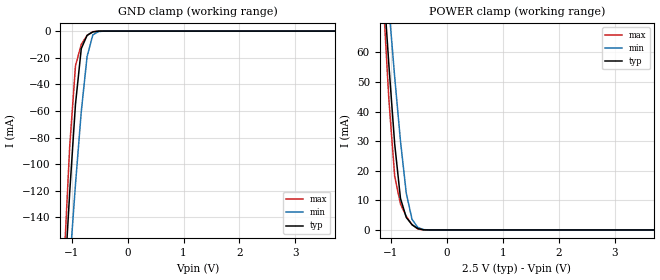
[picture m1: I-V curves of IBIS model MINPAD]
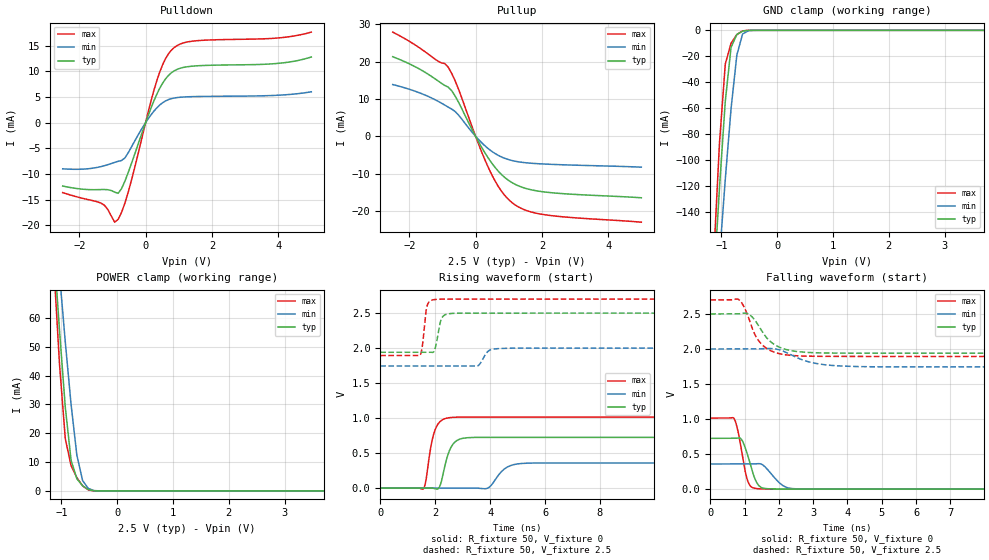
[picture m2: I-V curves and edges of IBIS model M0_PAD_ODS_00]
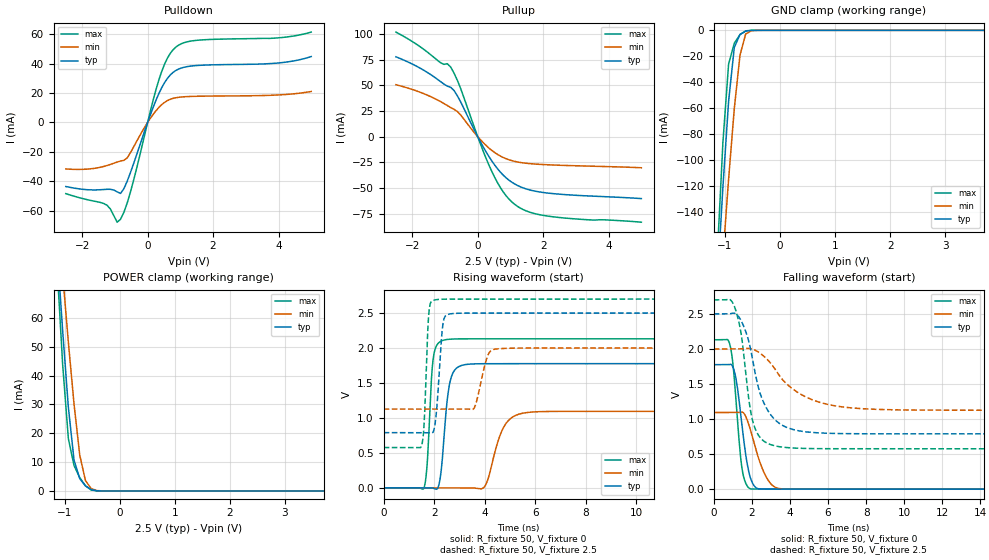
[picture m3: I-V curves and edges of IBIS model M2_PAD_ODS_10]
| Created by SiliconSmart  S-2021.06-SP5-2
[IBIS Ver]   4.0
[File Name]   as320ck_25v_rev1p1.ibs
[File Rev]   1.1
[Date]   Tue Aug 20 2024
|[Source]   Avalanche Team
|[Notes]   Generated IBIS models from Silicon Smart
|[Rev 1.0]   Initial release based on extracted netlist
|[Rev 1.1]   Updated the VCC supply values according to
|		datasheet
|[Disclaimer]   THE MODEL LIBRARIES ARE PROVIDED AS IS.
|[Copyright]   Copyright 2024, Avalanche Technology, All Rights Reserved
[Component]   AS30XX20X_BGA
[Manufacturer]  Avalanche Technology
| CONTENT :
| This file contains IBIS MODEL for PSRAM device
| AS30XX20X
| USAGE :
| The models are derived for the 2.0V to 2.7V I/O Operation.
| Temperatures for model generation: typ: 25, max: -40, min: 125
| Voltages : typ: 2.5V, min: 2.0V, max: 2.7V
| PACKAGES SUPPORTED :
| 56-ball FBGA (10mm x 10mm)
| VERIFICATION
| Errors  : 0
| Warnings: 11
| All warnings due to non-monotonic data:
[Package]
|  Design die-package: BGA
| variable   typ   min   max
R_pkg   0.72029   0.51528   1.0002
L_pkg   5.797e-9   4.155e-9   8.073e-9
C_pkg   1.116e-12   7.907e-13   1.753e-12
|Pin and Model info
[Pin]  signal_name  model_name   R_pin   L_pin   C_pin
E2   CS1#   MINPAD   0.4340	15.2000E-9	1.2600E-12
C3   CS2#   MINPAD   0.3800	13.5000E-9	1.0400E-12
D2   CLK1   MINPAD   0.4300	12.7000E-9	0.9790E-12
D1   CLK2   MINPAD   0.4480	14.6000E-9	1.1600E-12
F3   IO_0   MIOPAD   0.4010	12.4000E-9	1.2500E-12
F2   IO_1   MIOPAD   0.4050	14.2000E-9	1.1100E-12
E4   IO_2   MIOPAD   0.3780	11.8000E-9	1.2000E-12
F4   IO_3   MIOPAD   0.3700	11.8000E-9	1.2600E-12
F5   IO_4   MIOPAD   0.3710	11.1000E-9	1.1000E-12
G3   IO_5   MIOPAD   0.4050	13.8000E-9	1.1600E-12
G2   IO_6   MIOPAD   0.3830	15.2000E-9	1.0900E-12
G1   IO_7   MIOPAD   0.4480	16.4000E-9	1.0800E-12
C7   HTBSEL   MINPAD   0.1380	6.1700E-9	0.6060E-12
B7   HBP_2   MINPAD   0.1470	6.3900E-9	1.0000E-12
A6   HBP_1   MINPAD   0.1910	8.5000E-9	1.1500E-12
A5   HBP_0   MINPAD   0.2050	8.6800E-9	1.4200E-12
C4   RESET#   MINPAD   0.3410	14.1000E-9	1.6300E-12
C5   INT1#   MIOPAD   0.3080	12.5000E-9	1.2100E-12
D3   INT2#   MIOPAD   0.2120	10.3000E-9	0.8230E-12
B1   VSSIO   GND   NA   NA   NA
B5   VSSIO   GND   NA   NA   NA
B6   VSSIO   GND   NA   NA   NA
E1   VSSIO   GND   NA   NA   NA
G5   VSSIO   GND   NA   NA   NA
G6   VSSIO   GND   NA   NA   NA
A1   VSS   GND   NA   NA   NA
A3   VSS   GND   NA   NA   NA
B3   VSS   GND   NA   NA   NA
E5   VSS   GND   NA   NA   NA
E6   VSS   GND   NA   NA   NA
E7   VSS   GND   NA   NA   NA
G7   VSS   GND   NA   NA   NA
A8   VSS   GND   NA   NA   NA
A7   VCCIO   POWER   NA   NA   NA
B2   VCCIO   POWER   NA   NA   NA
B4   VCCIO   POWER   NA   NA   NA
C6   VCCIO   POWER   NA   NA   NA
F1   VCCIO   POWER   NA   NA   NA
F6   VCCIO   POWER   NA   NA   NA
G4   VCCIO   POWER   NA   NA   NA
A2   VCC   POWER   NA   NA   NA
A4   VCC   POWER   NA   NA   NA
D4   VCC   POWER   NA   NA   NA
D6   VCC   POWER   NA   NA   NA
D7   VCC   POWER   NA   NA   NA
F7   VCC   POWER   NA   NA   NA
| IOPAD
[Model Selector] MIOPAD
| Model Description
M0_PAD_ODS_00   35ohms
M1_PAD_ODS_01   40ohms
M2_PAD_ODS_10   20ohms
M3_PAD_ODS_11   15ohms
| Models and submodels in the file (5): MINPAD (Input), M0_PAD_ODS_00 (I/O), M2_PAD_ODS_10 (I/O), M1_PAD_ODS_01 (I/O), M3_PAD_ODS_11 (I/O)
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[Model] MINPAD
Model_type Input
Enable   Active-High
Vinl  =  0.7
Vinh  =  1.8
| Capacitance  typ   min   max
C_comp   1.561946e-12   1.465732e-12   1.706605e-12
| Variables   typ   min   max
[GND Clamp Reference]   0   0   0
[POWER Clamp Reference]   2.5   2   2.7
[Pulldown Reference]   0   0   0
[Pullup Reference]   2.5   2   2.7
[Temperature Range]   25   125   -40
[Voltage Range]   2.5   2   2.7
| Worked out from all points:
|   GND clamp passes 1 mA (typ) near -0.64 V on its own axis
|   POWER clamp passes 1 mA (typ) near -0.56 V on its own axis
[GND Clamp]
| Voltage   I(typ)   I(min)   I(max)
-2.5V     -1.297A    -1.146A    -1.538A
-1.138V   -195.9mA   -238.3mA   -175.2mA
-1.034V   -121.2mA   -175.1mA   -86.57mA
-931mV    -54.79mA   -114.9mA   -26.01mA
-827.6mV  -13.15mA   -60.41mA   -9.964mA
-724.1mV  -3.204mA   -19.15mA   -3.279mA
-620.7mV  -615.2uA   -2.798mA   -407.3uA
-517.2mV  -34.38uA   -319.4uA   -6.503uA
-413.8mV  -821.1nA   -24.43uA   -50.87nA
5V        0A         0A         0A
[POWER Clamp]
| Voltage   I(typ)   I(min)   I(max)
-2.5V     511mA      454.9mA    606.6mA
-1.138V   84.76mA    99.9mA     78.64mA
-1.034V   55.67mA    75.27mA    43.94mA
-931mV    29.07mA    51.7mA     18.16mA
-827.6mV  10.68mA    30.08mA    8.788mA
-724.1mV  4.238mA    12.45mA    4.618mA
-620.7mV  1.771mA    3.587mA    1.776mA
-517.2mV  465uA      837.9uA    329.7uA
-413.8mV  47.65uA    120.2uA    11.19uA
-310.3mV  1.515uA    11.72uA    116.8nA
5V        0A         0A         0A
[Model] M0_PAD_ODS_00
Model_type I/O
Enable   Active-High
Vinl  =  0.7
Vinh  =  1.8
Vmeas =  1.25
Cref  =  30e-12
| Capacitance  typ   min   max
C_comp   1.568193e-12   1.472592e-12   1.715469e-12
| Variables   typ   min   max
[GND Clamp Reference]   0   0   0
[POWER Clamp Reference]   2.5   2   2.7
[Pulldown Reference]   0   0   0
[Pullup Reference]   2.5   2   2.7
[Temperature Range]   25   125   -40
[Voltage Range]   2.5   2   2.7
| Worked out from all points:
|   slope of the pulldown table from 0 to 0.375 V, typ, clamps not added: 62.2 ohm
|   slope of the pullup table from 0 to 0.375 V, typ, clamps not added: 65.7 ohm
|   GND clamp passes 1 mA (typ) near -0.64 V on its own axis
|   POWER clamp passes 1 mA (typ) near -0.56 V on its own axis
|   falling waveform, R_fixture 50, V_fixture 0: 20-80 % time 278ps typ, 405ps min, 227ps max; typ from 0.725 V to 0 V
|   falling waveform, R_fixture 50, V_fixture 2.5: 20-80 % time 573ps typ, 848ps min, 480ps max; typ from 2.5 V to 1.94 V
|   rising waveform, R_fixture 50, V_fixture 0: 20-80 % time 317ps typ, 472ps min, 280ps max; typ from 0 V to 0.725 V
|   rising waveform, R_fixture 50, V_fixture 2.5: 20-80 % time 165ps typ, 246ps min, 130ps max; typ from 1.94 V to 2.5 V
[GND Clamp]
| Voltage   I(typ)   I(min)   I(max)
-2.5V     -1.297A    -1.146A    -1.538A
-1.138V   -195.9mA   -238.3mA   -175.2mA
-1.034V   -121.2mA   -175.1mA   -86.57mA
-931mV    -54.79mA   -114.9mA   -26.01mA
-827.6mV  -13.15mA   -60.41mA   -9.967mA
-724.1mV  -3.205mA   -19.15mA   -3.28mA
-620.7mV  -615.3uA   -2.798mA   -407.6uA
-517.2mV  -34.39uA   -319.4uA   -6.513uA
-413.8mV  -821.3nA   -24.43uA   -50.96nA
5V        0A         0A         0A
[POWER Clamp]
| Voltage   I(typ)   I(min)   I(max)
-2.5V     511mA      454.9mA    606.6mA
-1.138V   84.76mA    99.9mA     78.64mA
-1.034V   55.67mA    75.27mA    43.94mA
-931mV    29.07mA    51.7mA     18.16mA
-827.6mV  10.68mA    30.08mA    8.788mA
-724.1mV  4.238mA    12.45mA    4.618mA
-620.7mV  1.771mA    3.587mA    1.776mA
-517.2mV  465uA      837.9uA    329.7uA
-413.8mV  47.65uA    120.2uA    11.19uA
-310.3mV  1.515uA    11.72uA    116.8nA
5V        0A         0A         0A
[Pulldown]
| Voltage   I(typ)   I(min)   I(max)
-2.5V     -12.37mA   -9.009mA   -13.66mA
-1.345V   -13.05mA   -8.574mA   -15.7mA
-1.138V   -13.09mA   -8.194mA   -16.96mA
-931mV    -13.56mA   -7.743mA   -19.43mA
-827.6mV  -13.79mA   -7.541mA   -18.86mA
-517.2mV  -9.616mA   -5.796mA   -13.4mA
344.8mV   5.633mA    2.926mA    8.322mA
603.4mV   8.558mA    4.247mA    12.51mA
948.3mV   10.39mA    4.896mA    15.04mA
1.638V    11.13mA    5.111mA    16.04mA
3.99V     11.57mA    5.352mA    16.53mA
5V        12.82mA    6.029mA    17.68mA
[Pullup]
| Voltage   I(typ)   I(min)   I(max)
-2.5V     21.32mA    13.87mA    27.92mA
-1.552V   17.3mA     11.16mA    22.82mA
-827.6mV  13.18mA    7.828mA    18.54mA
-724.1mV  12.27mA    7.307mA    16.9mA
-517.2mV  9.182mA    5.729mA    12.71mA
86.21mV   -1.419mA   -832.2uA   -2.011mA
431mV     -6.452mA   -3.643mA   -9.245mA
775.9mV   -10.18mA   -5.508mA   -14.63mA
1.121V    -12.51mA   -6.533mA   -17.91mA
1.552V    -14.05mA   -7.116mA   -19.92mA
2.069V    -14.89mA   -7.424mA   -20.98mA
5V        -16.46mA   -8.263mA   -23mA
[Ramp]
dV/dt_r   0.434998/0.316698n  0.215611/0.472023n  0.608661/0.280321n
dV/dt_f   0.335983/0.573041n  0.153621/0.848322n  0.483841/0.48048n
R_load = 50
[Falling Waveform]
R_fixture = 50
V_fixture = 0
V_fixture_min = 0
V_fixture_max = 0
| Time   V(typ)   V(min)   V(max)
0s        725mV      359.4mV    1.014V
692.7ps   725.4mV    359.9mV    1.009V
780.7ps   727.4mV    359.9mV    883.5mV
897.1ps   717.9mV    360mV      593.3mV
1.087ns   490mV      360.1mV    124.4mV
1.367ns   83.45mV    363.9mV    7.307mV
1.567ns   12.57mV    331.9mV    2.275mV
2.126ns   1.009mV    48.03mV    266.1uV
2.527ns   365uV      4.584mV    159.6uV
21.88ns   -231.7nV   204.9nV    -107.4nV
[Falling Waveform]
R_fixture = 50
V_fixture = 2.5
V_fixture_min = 2
V_fixture_max = 2.7
| Time   V(typ)   V(min)   V(max)
0s        2.5V       2V         2.7V
823.1ps   2.501V     2.001V     2.707V
1.153ns   2.487V     2.001V     2.396V
1.304ns   2.409V     2.001V     2.203V
1.519ns   2.246V     2.004V     2.057V
1.886ns   2.058V     2.002V     1.951V
2.393ns   1.974V     1.908V     1.907V
3.087ns   1.946V     1.793V     1.895V
4.331ns   1.94V      1.749V     1.894V
21.88ns   1.94V      1.744V     1.894V
[Rising Waveform]
R_fixture = 50
V_fixture = 0
V_fixture_min = 0
V_fixture_max = 0
| Time   V(typ)   V(min)   V(max)
0s        3.584nV    84.08nV    3.3nV
1.569ns   -28.5uV    -123.8uV   -11.33mV
1.991ns   -8.017mV   -157.2uV   826.6mV
2.178ns   36.02mV    -171.9uV   950mV
2.497ns   512.7mV    -197.1uV   1.005V
2.897ns   699.7mV    -228.7uV   1.013V
3.862ns   724.3mV    -7.558mV   1.014V
4.611ns   724.4mV    297.4mV    1.014V
5.389ns   724.4mV    356.4mV    1.014V
21.88ns   725mV      359.4mV    1.014V
[Rising Waveform]
R_fixture = 50
V_fixture = 2.5
V_fixture_min = 2
V_fixture_max = 2.7
| Time   V(typ)   V(min)   V(max)
0s        1.94V      1.744V     1.894V
1.451ns   1.941V     1.744V     1.898V
1.701ns   1.941V     1.744V     2.597V
2.038ns   2.059V     1.745V     2.695V
2.245ns   2.432V     1.745V     2.699V
2.653ns   2.496V     1.745V     2.699V
3.54ns    2.499V     1.745V     2.699V
3.956ns   2.499V     1.964V     2.699V
4.503ns   2.499V     1.996V     2.699V
21.88ns   2.5V       2V         2.7V
[Model] M2_PAD_ODS_10
Model_type I/O
Enable   Active-High
Vinl  =  0.7
Vinh  =  1.8
Vmeas =  1.25
Cref  =  30e-12
| Capacitance  typ   min   max
C_comp   1.568193e-12   1.472592e-12   1.715469e-12
| Variables   typ   min   max
[GND Clamp Reference]   0   0   0
[POWER Clamp Reference]   2.5   2   2.7
[Pulldown Reference]   0   0   0
[Pullup Reference]   2.5   2   2.7
[Temperature Range]   25   125   -40
[Voltage Range]   2.5   2   2.7
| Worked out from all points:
|   slope of the pulldown table from 0 to 0.375 V, typ, clamps not added: 17.8 ohm
|   slope of the pullup table from 0 to 0.375 V, typ, clamps not added: 18 ohm
|   GND clamp passes 1 mA (typ) near -0.64 V on its own axis
|   POWER clamp passes 1 mA (typ) near -0.56 V on its own axis
|   falling waveform, R_fixture 50, V_fixture 0: 20-80 % time 505ps typ, 778ps min, 385ps max; typ from 1.78 V to 0 V
|   falling waveform, R_fixture 50, V_fixture 2.5: 20-80 % time 1.03ns typ, 2.06ns min, 615ps max; typ from 2.5 V to 0.789 V
|   rising waveform, R_fixture 50, V_fixture 0: 20-80 % time 269ps typ, 559ps min, 183ps max; typ from 0 V to 1.78 V
|   rising waveform, R_fixture 50, V_fixture 2.5: 20-80 % time 193ps typ, 337ps min, 136ps max; typ from 0.789 V to 2.5 V
[GND Clamp]
| Voltage   I(typ)   I(min)   I(max)
-2.5V     -1.297A    -1.146A    -1.538A
-1.138V   -195.9mA   -238.3mA   -175.2mA
-1.034V   -121.2mA   -175.1mA   -86.57mA
-931mV    -54.79mA   -114.9mA   -26.01mA
-827.6mV  -13.15mA   -60.41mA   -9.967mA
-724.1mV  -3.205mA   -19.15mA   -3.28mA
-620.7mV  -615.3uA   -2.798mA   -407.6uA
-517.2mV  -34.39uA   -319.4uA   -6.513uA
-413.8mV  -821.3nA   -24.43uA   -50.96nA
5V        0A         0A         0A
[POWER Clamp]
| Voltage   I(typ)   I(min)   I(max)
-2.5V     511mA      454.9mA    606.6mA
-1.138V   84.76mA    99.9mA     78.64mA
-1.034V   55.67mA    75.27mA    43.94mA
-931mV    29.07mA    51.7mA     18.16mA
-827.6mV  10.68mA    30.08mA    8.788mA
-724.1mV  4.238mA    12.45mA    4.618mA
-620.7mV  1.771mA    3.587mA    1.776mA
-517.2mV  465uA      837.9uA    329.7uA
-413.8mV  47.65uA    120.2uA    11.19uA
-310.3mV  1.515uA    11.72uA    116.8nA
5V        0A         0A         0A
[Pulldown]
| Voltage   I(typ)   I(min)   I(max)
-2.5V     -43.54mA   -31.62mA   -48.38mA
-1.345V   -45.58mA   -29.95mA   -55.04mA
-1.138V   -45.44mA   -28.55mA   -58.81mA
-931mV    -47.17mA   -26.91mA   -67.8mA
-827.6mV  -48.24mA   -26.21mA   -65.83mA
-517.2mV  -33.61mA   -20.26mA   -46.69mA
344.8mV   19.68mA    10.22mA    29mA
603.4mV   29.91mA    14.84mA    43.66mA
948.3mV   36.32mA    17.11mA    52.56mA
1.638V    38.89mA    17.86mA    56.1mA
3.99V     40.44mA    18.69mA    57.52mA
5V        44.82mA    21.06mA    61.44mA
[Pullup]
| Voltage   I(typ)   I(min)   I(max)
-2.5V     77.66mA    50.55mA    101.7mA
-1.552V   62.71mA    40.56mA    82.54mA
-1.138V   53.61mA    34.15mA    71.93mA
-827.6mV  48.08mA    28.39mA    67.76mA
-517.2mV  33.57mA    20.94mA    46.41mA
86.21mV   -5.185mA   -3.042mA   -7.343mA
431mV     -23.58mA   -13.31mA   -33.77mA
775.9mV   -37.21mA   -20.13mA   -53.46mA
1.121V    -45.74mA   -23.87mA   -65.48mA
1.552V    -51.37mA   -26mA      -72.89mA
2.155V    -54.78mA   -27.26mA   -77.18mA
5V        -60.09mA   -30.14mA   -83.02mA
[Ramp]
dV/dt_r   1.06541/0.26881n  0.65595/0.55939n  1.27868/0.183118n
dV/dt_f   1.02665/1.03344n  0.524479/2.05985n  1.27424/0.615015n
R_load = 50
[Falling Waveform]
R_fixture = 50
V_fixture = 0
V_fixture_min = 0
V_fixture_max = 0
| Time   V(typ)   V(min)   V(max)
0s        1.776V     1.093V     2.131V
853.4ps   1.78V      1.094V     2.054V
997.5ps   1.746V     1.094V     1.808V
1.167ns   1.575V     1.094V     1.266V
1.457ns   968.2mV    1.099V     345.3mV
1.616ns   613.4mV    1.069V     129.8mV
1.903ns   181mV      866.8mV    7.495mV
2.701ns   2.004mV    201.7mV    764.5uV
3.407ns   915.4uV    9.526mV    418uV
21.88ns   -194.7nV   403.6pV    -423.4nV
[Falling Waveform]
R_fixture = 50
V_fixture = 2.5
V_fixture_min = 2
V_fixture_max = 2.7
| Time   V(typ)   V(min)   V(max)
0s        2.5V       2V         2.7V
1.078ns   2.51V      2V         2.613V
1.422ns   2.413V     2.001V     2.242V
1.827ns   2.119V     2.008V     1.309V
2.055ns   1.828V     1.995V     959.7mV
2.453ns   1.35V      1.936V     730mV
2.999ns   1.057V     1.793V     633.9mV
4.478ns   831.9mV    1.369V     583.4mV
6.697ns   792.9mV    1.175V     576.6mV
21.88ns   788.9mV    1.126V     576.3mV
[Rising Waveform]
R_fixture = 50
V_fixture = 0
V_fixture_min = 0
V_fixture_max = 0
| Time   V(typ)   V(min)   V(max)
0s        2.114nV    46.37nV    1.824nV
1.601ns   -420uV     -435.4uV   523.8uV
1.97ns    -7.665mV   -535.7uV   1.865V
2.378ns   659.2mV    -646.7uV   2.113V
2.653ns   1.55V      -721.3uV   2.127V
3.242ns   1.763V     -881.5uV   2.131V
4.009ns   1.775V     21.73mV    2.131V
4.727ns   1.776V     847.2mV    2.131V
5.515ns   1.776V     1.067V     2.131V
21.88ns   1.776V     1.093V     2.131V
[Rising Waveform]
R_fixture = 50
V_fixture = 2.5
V_fixture_min = 2
V_fixture_max = 2.7
| Time   V(typ)   V(min)   V(max)
0s        788.9mV    1.126V     576.3mV
1.497ns   788.5mV    1.126V     597.7mV
1.602ns   788.5mV    1.126V     906.9mV
1.792ns   788.5mV    1.126V     2.506V
2.019ns   873.8mV    1.126V     2.687V
2.333ns   2.298V     1.127V     2.698V
2.591ns   2.485V     1.127V     2.699V
3.564ns   2.499V     1.13V      2.699V
4.436ns   2.499V     1.985V     2.699V
21.88ns   2.5V       2V         2.7V
